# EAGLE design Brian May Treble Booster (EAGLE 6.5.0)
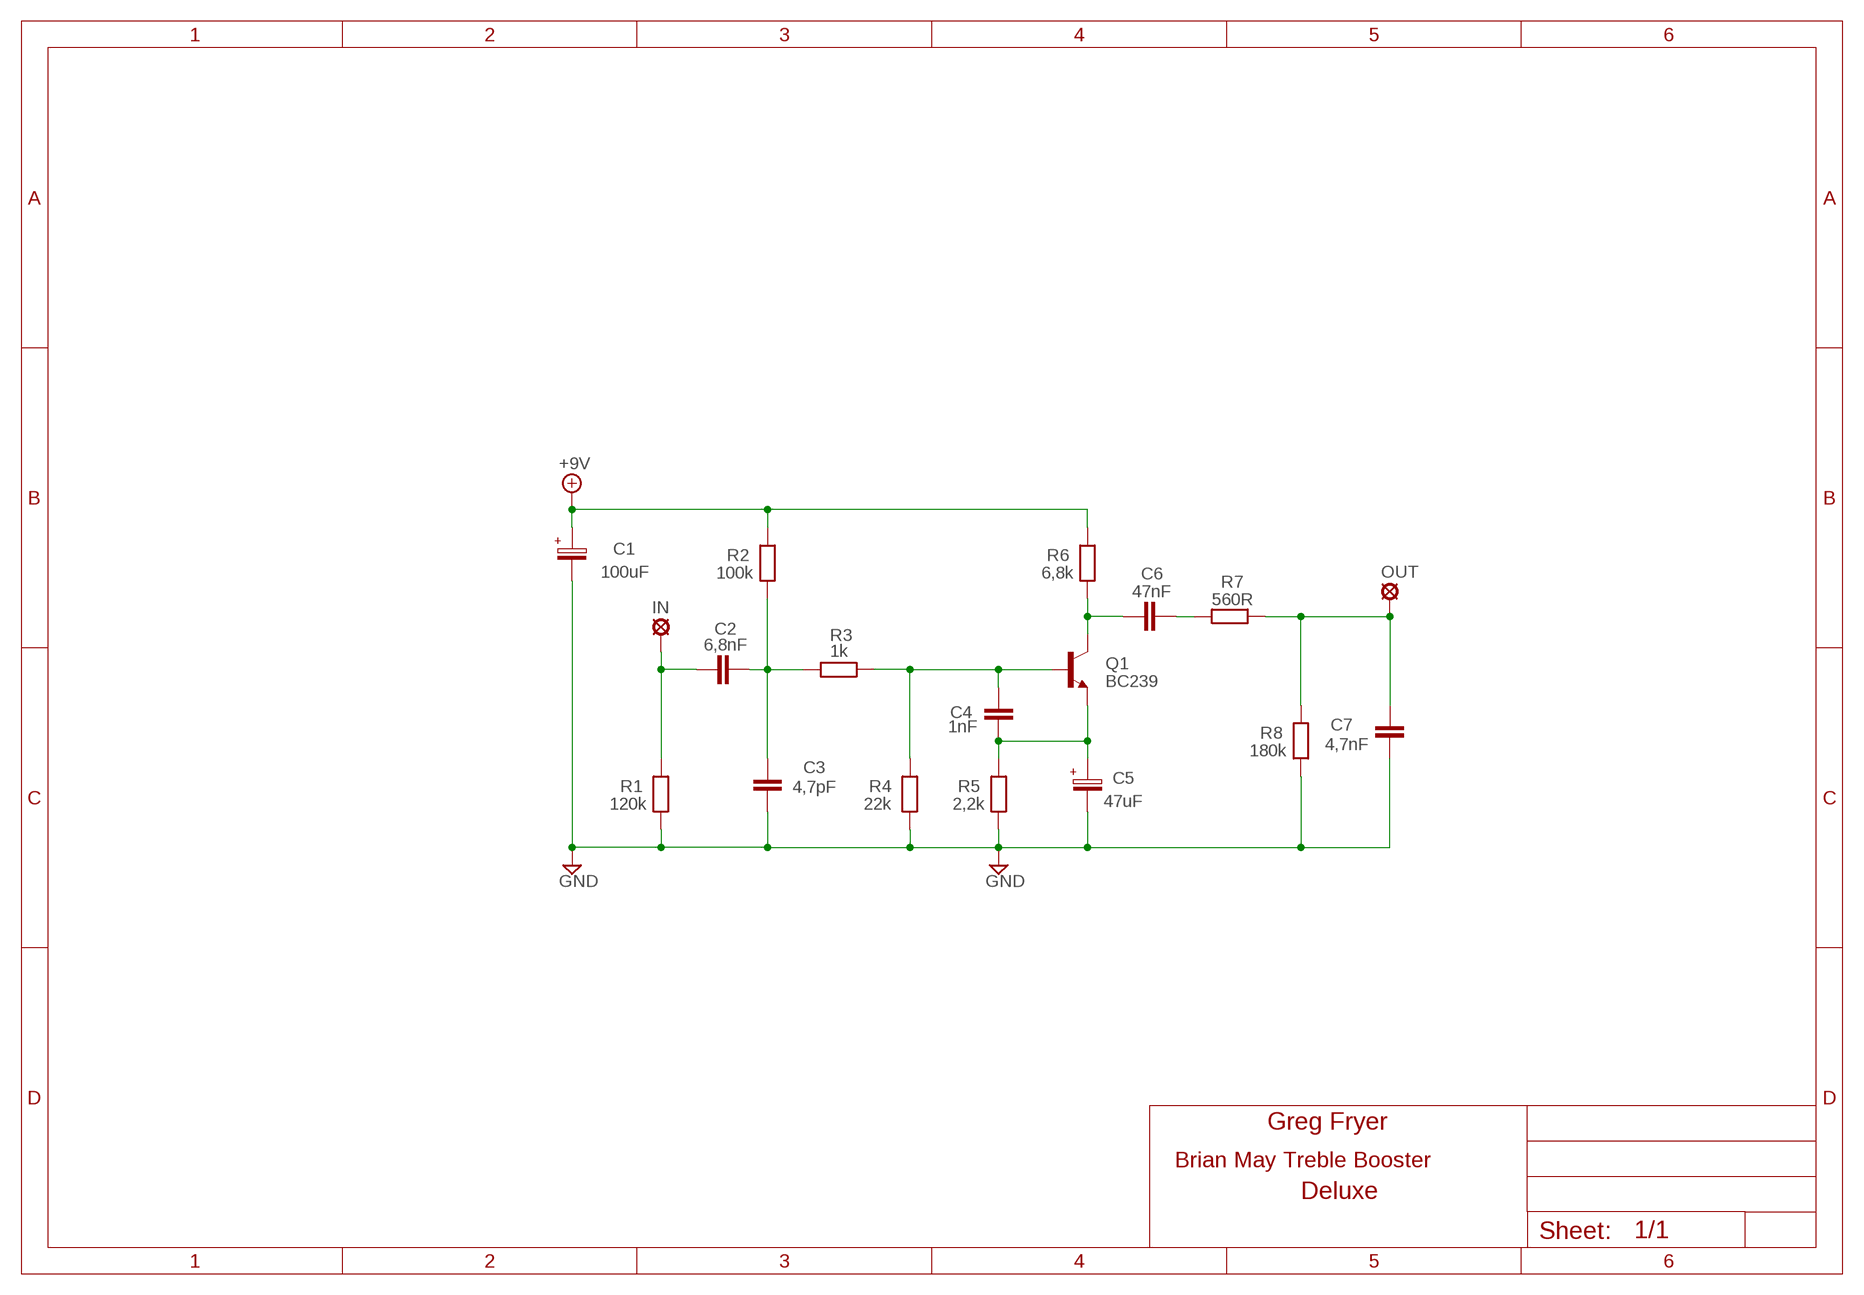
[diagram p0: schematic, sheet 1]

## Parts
+9V  +9V  +9V(T)1  [ROUND]
C1  100uF  063-EU  [063_025]
C2  6,8nF  1NF-15NF  [3,5MM]
C3  4,7pF  050X030_0252  [050X030_025_2]
C4  1nF  1NF-15NF  [3,5MM]
C5  47uF  063-EU  [063_025]
C6  47nF  22NF-82NF"  [4,5MM]
C7  4,7nF  1NF-15NF  [3,5MM]
GND  GND  GND(T)1  [ROUND]
GND1  GND  GND(T)1  [ROUND]
IN  MCS10B  [MCS10B]
OUT  MCS10B  [MCS10B]
Q1  BC239  [TO92]
R1  120k  6MM-EU3  [R0207/3]
R2  100k  6MM-EU3  [R0207/3]
R3  1k  6MM-EU3  [R0207/3]
R4  22k  6MM-EU3  [R0207/3]
R5  2,2k  6MM-EU3  [R0207/3]
R6  6,8k  6MM-EU3  [R0207/3]
R7  560R  6MM-EU3  [R0207/3]
R8  180k  6MM-EU3  [R0207/3]

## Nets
+9V: +9V.1(+9V) C1.+ R2.2 R6.2
GND: C1.- C3.2 C5.- C7.1 GND1.1(GND) GND.1(GND) R1.1 R4.1 R5.1 R8.1
N$1: C2.1 IN.MP R1.2
N$2: C2.2 C3.1 R2.1 R3.1
N$4: C4.2 Q1.2(B) R3.2 R4.2
N$5: C6.1 Q1.3(C) R6.1
N$6: C6.2 R7.1
N$7: C7.2 OUT.MP R7.2 R8.2
N$8: C4.1 C5.+ Q1.1(E) R5.2

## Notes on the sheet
- Greg Fryer
- Deluxe

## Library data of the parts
+9V = gm-supply:+9V(T): +9V Voltage Supply
C1 C5 = Elektrolyytit:063-EU
C2 C4 C7 = Mylar Kondensaattorit:1NF-15NF: 1nF-15nF
C3 = Keraamiset kondensaattorit:050X030_025: 47 - 120pF
C6 = Mylar Kondensaattorit:22NF-82NF: 22nF-82nF
GND GND1 = gm-supply:GND(T): Ground
IN OUT = Padit:MCS10B: SOLDER PAD
Q1 = Transistorit:BC239: NPN Transistor
R1-R8 = Vastukset:6MM-EU: 6mm Resistors (European schematic symbol)

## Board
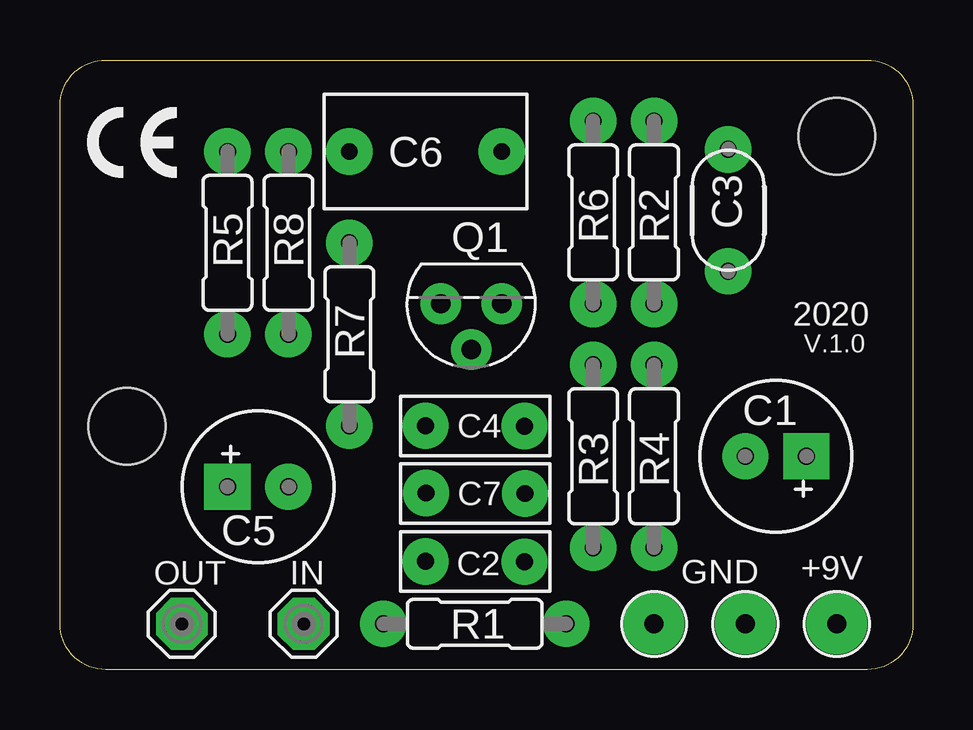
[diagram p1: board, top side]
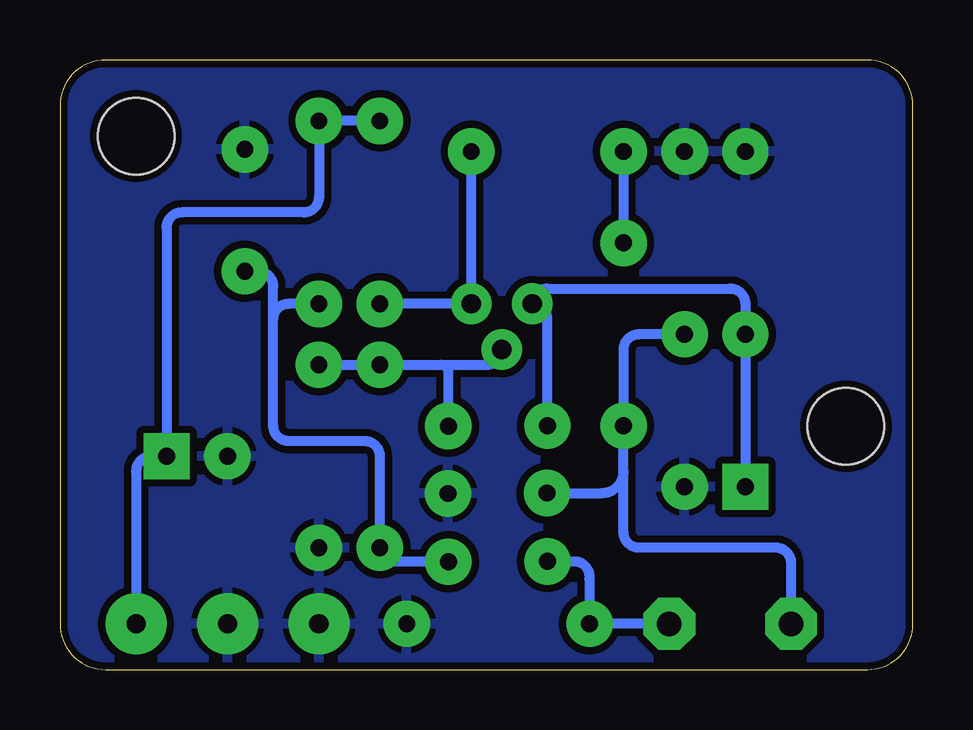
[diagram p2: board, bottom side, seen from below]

Size 35.56 x 25.4 mm. Coordinates in mm from the lower left corner, seen from the top.
Outline: 1.91,25.4 33.66,25.4 arc-90 35.56,23.5 35.56,1.91 arc-90 33.66,0 1.91,0 arc-90 0,1.91 0,23.5 arc-90 1.91,25.4
Copper layers (1*16): Top 0.035mm / dielectric 1.5mm / Bottom 0.035mm
Design rules "ITEADstudio": minimum track width 10mil, minimum drill 12mil, track to track 12mil, track to pad 12mil, pad to pad 12mil, via to via 12mil, smd to smd 0mil, copper to edge 12mil, drill to drill 12mil, minimum pad ring 10mil, minimum via ring 6mil, stop-mask expansion 4mil, vias tented up to drill 100mil, thermal gap 10mil
Holes 3.2 mm at 32.38,22.23 2.8,10.14

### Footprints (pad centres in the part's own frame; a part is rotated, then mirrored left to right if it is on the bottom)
ROUND = drill 0.8 pad 2.54: 1 0,0
063_025 = drill 0.7 pad 1.93 square: + -1.27,0 | drill 0.7 pad 1.93: - 1.27,0
3,5MM = drill 0.7 pad 1.93: 1 -1.905,0; 2 2.221,-0.016
050X030_025_2 = drill 0.7 pad 1.93: 1 -2.54,0; 2 2.54,0
4,5MM = drill 0.7 pad 1.93: 1 -3.175,0; 2 3.175,0
MCS10B = drill 1.016 pad 2.159 octagon: MP 0,0
TO92 = drill 0.8 pad 1.7: 1 1.27,0; 2 0,1.905; 3 -1.27,0
R0207/3 = drill 0.7 pad 1.93: 1 -3.81,0; 2 3.81,0

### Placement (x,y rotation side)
+9V  32.38,1.91 0 top
C1  29.84,8.89 180 top
C2  17.14,4.51 0 top
C3  27.86,19.14 90 top
C4  17.14,10.16 0 top
C5  8.26,7.62 0 top
C6  15.24,21.59 180 top
C7  17.48,7.34 180 top
GND  24.77,1.91 0 top
GND1  28.57,1.91 0 top
IN  10.16,1.91 0 top
OUT  5.08,1.91 0 top
Q1  17.14,15.24 180 top
R1  17.29,1.91 180 top
R2  24.77,19.05 90 top
R3  22.23,8.89 90 top
R4  24.77,8.89 90 top
R5  6.99,17.78 270 top
R6  22.23,19.05 90 top
R7  12.06,13.97 270 top
R8  9.53,17.78 270 top

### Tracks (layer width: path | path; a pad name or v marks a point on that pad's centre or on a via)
+9V
  Bottom 0.406: R6.2 R2.2 24.77,19.68 arc90 25.4,19.05 30.48,19.05 arc-90 31.11,18.41 C1.+ 31.75,8.89 arc-90 32.38,8.26 +9V.1
GND
  pour Bottom: 0,2.54 0,22.86 arc-90 1.91,25.4 33.66,25.4 arc-90 35.56,22.86 35.56,1.91 arc-90 33.66,0 1.27,0 arc-90
N$1
  Bottom 0.406: IN.MP R1.2 arc90 R1.2 arc-90 13.49,2.02 13.49,3.78 arc-90 14.04,4.51 C2.1
N$2
  Bottom 0.406: C3.1 27.3,16.6 arc90 26.67,15.96 26.67,14.61 | 26.67,14.61 26.67,10.16 arc-90 26.04,9.53 22.86,9.53 arc90 22.23,8.89 R3.1 arc-90 21.64,4.49 C2.2 | R2.1 26.04,15.24 arc-90 26.67,14.61
N$4
  Bottom 0.406: R4.2 R3.2 19.68,12.7 | 19.68,12.7 17.78,12.7 arc-90 Q1.2 | C4.2 19.37,12.38 arc-90 19.68,12.7
N$5
  Bottom 0.406: C6.1 Q1.3 R6.1
N$6
  Bottom 0.406: C6.2 R7.1
N$7
  Bottom 0.406: C7.2 12.96,7.36 arc-90 12.06,8.26 | 12.06,8.26 R7.2 12.06,13.34 arc90 11.43,13.97 R8.2 | OUT.MP 5.08,4.45 arc-90 5.71,5.08 11.43,5.08 arc90 12.06,5.71 12.06,8.26
N$8
  Bottom 0.406: C5.+ R5.2 6.99,15.24 arc-90 7.62,15.88 15.24,15.88 arc-90 Q1.1 arc90 15.24,14.61 C4.1

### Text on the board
tNames: 2020 | V.1.0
